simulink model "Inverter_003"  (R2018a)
settings: Solver=FixedStepDiscrete  StartTime=0.0  StopTime=inf  RelTol=1e-3  EnableMultiTasking=on
PreLoadFcn:
  | Sample_Time
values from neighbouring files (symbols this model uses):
  C_filt = 4.7e-6 /2  /2    (= 1.175e-06)    [Sample_Time.m]
  L_filt = 10e-3  /2  *2    (= 0.01)    [Sample_Time.m]
  Tcontrol = 5e-5    (= 5e-05)    [Sample_Time.m]
  Tmeasure = 5e-5     *2    (= 0.0001)    [Sample_Time.m]
  Tsample = 1e-6    (= 1e-06)    [Sample_Time.m]
  Tscope = Tcontrol*20    (= 0.001)    [Sample_Time.m]
  w = 2*pi*50    (= 314.159265359)    [Sample_Time.m]
undefined symbols (not defined in the file or in its folder): A, ADCIN0, ADCIN1, ADCINA0, ADCINB0, bit, C_filtEST, Compare, conversion, DCAEVT1, DCAEVT1FILT, Digital, Down, ended, Event, Filtered, GPTRIP1SEL, GPTRIP2SEL, input, Module, of, Single, start, Trip, TZ1, TZ2, Up, version, Zone
libraries: tiiqmathlib x32, simulink x16, c2802xlib x13, c2837xDlib x13, powerlib_meascontrol x4, etargetslib x4, c28xdmclib x1
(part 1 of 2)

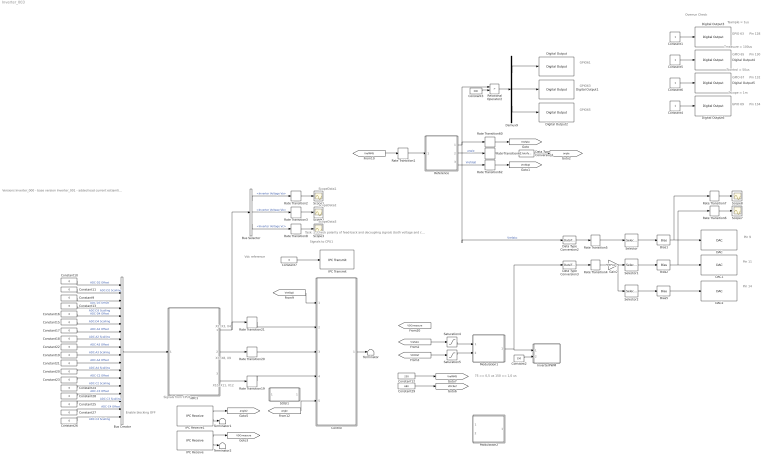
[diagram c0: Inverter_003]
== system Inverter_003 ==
  note: X2, X3, X4
  note: ScopeData3
  note: ScopeData2
  note: ScopeData1
  note: Vdc reference
  note: Enable blocking OFF
  note: Versions Inverter_000 - base version Inverter_001 - added load current estiamtion in control block Inverter_002 - PIR controller same as in PhD simulations Inverter_003 - Major changes to scaling and control blocks
  note: Task: 1. Check polarity of feed-back and decoupling signals (both voltage and current control)
  note: 75 == 0,5 us 150 == 1,0 us
  note: GPIO61
  note: GPIO63
  note: GPIO65
  note: Tcontrol = 50us
  note: GPIO 63
  note: Overrun Check
  note: Pin 128
  note: GPIO 69
  note: Pin 130
  note: Pin 134
  note: Pin 132
  note: GPIO 65
  note: Tsample = 1us
  note: Tmeasure = 100us
  note: Tscope = 1m
  note: GPIO 67
  note: Pin 14
  note: Pin 9
  note: Pin 11
  note: Signals from CPU1
  note: Signals to CPU1
  note: X7, X8, X9
  note: X10, X11, X12
  ADC1 : Subsystem
  Bias1 : Bias  Bias=400
  Bias2 : Bias  Bias=400
  Bias5 : Bias  Bias=400
  Bus Creator : BusCreator  Inputs=18
  Bus Selector : BusSelector  OutputSignals=Inverter Voltage Va,Inverter Voltage Vb,Inverter Voltage Vc
  Constant1 : Constant  Commented=on  SampleTime=Tsample
  Constant{9..11,13,15..28} (18 alike) : Constant  Value=0  OutDataTypeStr=single  SampleTime=0.1
  Constant12 : Constant  Value=230  OutDataTypeStr=single  SampleTime=0.1
  Constant2 : Constant  Value=150  OutDataTypeStr=single  SampleTime=0.1
  Constant29 : Constant  Value=680  OutDataTypeStr=fixdt(1,32,2^-10,0)  SampleTime=0.1
  Constant3 : Constant  Value=300  OutDataTypeStr=fixdt(1,32,2^-10,0)  SampleTime=0.1
  Constant4 : Constant  SampleTime=Tscope
  Constant5 : Constant  SampleTime=Tmeasure
  Constant6 : Constant  SampleTime=Tcontrol
  Constant7 : Constant  Value=0  OutDataTypeStr=single  SampleTime=Tcontrol
  Control : Subsystem  Commented=on
  DAC : c2837xDlib/DAC  channel=A  saturate=off
  DAC1 : c2837xDlib/DAC  channel=B  saturate=off
  DAC2 : c2837xDlib/DAC  channel=C  saturate=off
  Data Type Conversion1 : DataTypeConversion  OutDataTypeStr=single
  Data Type Conversion2 : DataTypeConversion  OutDataTypeStr=single
  Data Type Conversion3 : DataTypeConversion  OutDataTypeStr=single
  Demux9 : Demux  Outputs=3
  Digital Output : c2837xDlib/Digital Output  GPIO_Number=GPIO56~GPIO63  GPIO_Bit0=off  GPIO_BIT0_Toggle=off  GPIO_Bit1=off  GPIO_BIT1_Toggle=off  GPIO_Bit2=off  GPIO_BIT2_Toggle=off  GPIO_Bit3=off  GPIO_BIT3_Toggle=off  GPIO_Bit4=off  GPIO_BIT4_Toggle=off  GPIO_Bit5=on  GPIO_BIT5_Toggle=off  GPIO_Bit6=off  GPIO_BIT6_Toggle=off  GPIO_Bit7=off  GPIO_BIT7_Toggle=off
  Digital Output1 : c2837xDlib/Digital Output  GPIO_Number=GPIO56~GPIO63  GPIO_Bit0=off  GPIO_BIT0_Toggle=off  GPIO_Bit1=off  GPIO_BIT1_Toggle=off  GPIO_Bit2=off  GPIO_BIT2_Toggle=off  GPIO_Bit3=off  GPIO_BIT3_Toggle=off  GPIO_Bit4=off  GPIO_BIT4_Toggle=off  GPIO_Bit5=off  GPIO_BIT5_Toggle=off  GPIO_Bit6=off  GPIO_BIT6_Toggle=off  GPIO_Bit7=on  GPIO_BIT7_Toggle=off
  Digital Output2 : c2837xDlib/Digital Output  GPIO_Number=GPIO64~GPIO71  GPIO_Bit0=off  GPIO_BIT0_Toggle=off  GPIO_Bit1=off  GPIO_BIT1_Toggle=off  GPIO_Bit2=on  GPIO_BIT2_Toggle=off  GPIO_Bit3=off  GPIO_BIT3_Toggle=off  GPIO_Bit4=off  GPIO_BIT4_Toggle=off  GPIO_Bit5=off  GPIO_BIT5_Toggle=off  GPIO_Bit6=off  GPIO_BIT6_Toggle=off  GPIO_Bit7=off  GPIO_BIT7_Toggle=off
  Digital Output3 : c2837xDlib/Digital Output  Commented=on  GPIO_Number=GPIO56~GPIO63  GPIO_Bit0=off  GPIO_BIT0_Toggle=on  GPIO_Bit1=off  GPIO_BIT1_Toggle=off  GPIO_Bit2=off  GPIO_BIT2_Toggle=on  GPIO_Bit3=off  GPIO_BIT3_Toggle=off  GPIO_Bit4=off  GPIO_BIT4_Toggle=off  GPIO_Bit5=off  GPIO_BIT5_Toggle=off  GPIO_Bit6=off  GPIO_BIT6_Toggle=off  GPIO_Bit7=on  GPIO_BIT7_Toggle=on
  Digital Output4 : c2837xDlib/Digital Output  GPIO_Number=GPIO64~GPIO71  GPIO_Bit0=off  GPIO_BIT0_Toggle=on  GPIO_Bit1=on  GPIO_BIT1_Toggle=on  GPIO_Bit2=off  GPIO_BIT2_Toggle=on  GPIO_Bit3=off  GPIO_BIT3_Toggle=off  GPIO_Bit4=off  GPIO_BIT4_Toggle=off  GPIO_Bit5=off  GPIO_BIT5_Toggle=off  GPIO_Bit6=off  GPIO_BIT6_Toggle=off  GPIO_Bit7=off  GPIO_BIT7_Toggle=off
  Digital Output5 : c2837xDlib/Digital Output  GPIO_Number=GPIO64~GPIO71  GPIO_Bit0=off  GPIO_BIT0_Toggle=off  GPIO_Bit1=off  GPIO_BIT1_Toggle=off  GPIO_Bit2=off  GPIO_BIT2_Toggle=on  GPIO_Bit3=on  GPIO_BIT3_Toggle=on  GPIO_Bit4=off  GPIO_BIT4_Toggle=off  GPIO_Bit5=off  GPIO_BIT5_Toggle=off  GPIO_Bit6=off  GPIO_BIT6_Toggle=off  GPIO_Bit7=off  GPIO_BIT7_Toggle=off
  Digital Output6 : c2837xDlib/Digital Output  GPIO_Number=GPIO64~GPIO71  GPIO_Bit0=off  GPIO_BIT0_Toggle=on  GPIO_Bit1=off  GPIO_BIT1_Toggle=off  GPIO_Bit2=off  GPIO_BIT2_Toggle=on  GPIO_Bit3=off  GPIO_BIT3_Toggle=on  GPIO_Bit4=off  GPIO_BIT4_Toggle=off  GPIO_Bit5=on  GPIO_BIT5_Toggle=on  GPIO_Bit6=off  GPIO_BIT6_Toggle=off  GPIO_Bit7=off  GPIO_BIT7_Toggle=off
  Gain2 : Gain  Gain=230*sqrt(2)
  IPC Receive : c2837xDlib/IPC Receive  SelectChannel=0  DataType=single  DataLength=1  EnableBlocking=off  SampleTime=Tcontrol
  IPC Receive1 : c2837xDlib/IPC Receive  SelectChannel=2  DataType=single  DataLength=1  EnableBlocking=off  SampleTime=Tcontrol
  IPC Transmit : c2837xDlib/IPC Transmit  SelectChannel=1  EnableBlocking=off
  InverterPWM : Subsystem
  Modulation1 : Subsystem
  Modulation2 : Subsystem  Commented=on
  Rate Transition1 : RateTransition  OutPortSampleTime=10e-5
  Rate Transition{4..5,19..21,60..62} (8 alike) : RateTransition  OutPortSampleTime=Tcontrol
  Rate Transition2 : RateTransition  OutPortSampleTime=Tscope
  Rate Transition3 : RateTransition  OutPortSampleTime=Tscope
  Rate Transition6 : RateTransition  Commented=on  OutPortSampleTime=Tscope
  Rate Transition7 : RateTransition  Commented=on  OutPortSampleTime=Tscope
  Rate Transition8 : RateTransition  OutPortSampleTime=Tscope
  Reference : Subsystem  Commented=on
  Relational Operator2 : RelationalOperator  Operator=>  OutDataTypeStr=boolean
  SOGI1 : Subsystem  Commented=on  TreatAsAtomicUnit=on  mask{Freq=50, SampleTime=Tcontrol, UpperLimit=1000, LowerLimit=-1000}
      mask prompts: Freq "Frequency, Hz"; SampleTime "Sample Time, s"; UpperLimit "Upper Limit"; LowerLimit "Lower Limit"
  Saturation4 : Saturate  UpperLimit=400  LowerLimit=-400
  Saturation5 : Saturate  UpperLimit=720  LowerLimit=0
  Scope{1..3,7..8} (5 alike) : Scope
  Selector : Selector  InputPortWidth=3  IndexOptions=Index vector (dialog)  Indices=[2]  OutputSizes=1
  Selector1 : Selector  InputPortWidth=4  IndexOptions=Index vector (dialog)  Indices=[2]  OutputSizes=1
  Selector2 : Selector  InputPortWidth=4  IndexOptions=Index vector (dialog)  Indices=[4]  OutputSizes=1
  Terminator : Terminator
  Terminator1 : Terminator
  Terminator2 : Terminator
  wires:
  [Vrefabc] -> Saturation4/1
  [angle] -> Control/5(Angle)
  Constant2/1 -> InverterPWM/2(DeadBand)
  Saturation4/1 -> Modulation1/1(Vcontrol)
  Modulation1/1(VPWM) -> Data Type Conversion3/1, InverterPWM/1(PWM)
  Saturation5/1 -> Modulation1/2(VDC)
  Rate Transition21/1 -> Control/2(Vabc Phase)
  [Vrefdq0] -> Control/1(dq0Ref)
  [VDCRef] -> Saturation5/1
  Control/1(Vabc Control) -> Terminator/1
  Rate Transition20/1 -> Control/3(Iabc Inv)
  Rate Transition19/1 -> Control/4(Iabc Load)
  Demux9/2 -> Digital Output1/1
  Rate Transition1/1 -> Reference/1(Vac Ref)
  [VrefRMS] -> Rate Transition1/1
  Rate Transition61/1 -> Data Type Conversion1/1
  Reference/3(dq0) -> Rate Transition62/1  "Vrefdq0"
  Rate Transition62/1 -> [Vrefdq0]
  Reference/1(abc) -> Data Type Conversion2/1, Relational Operator2/1, Rate Transition60/1  "Vrefabc"
  Demux9/3 -> Digital Output2/1
  Reference/2(angle) -> Rate Transition61/1  "angle"
  Rate Transition60/1 -> [Vrefabc]
  Demux9/1 -> Digital Output/1
  Relational Operator2/1 -> Demux9/1
  Constant3/1 -> Relational Operator2/2
  Rate Transition4/1 -> Gain2/1
  Rate Transition5/1 -> Selector/1
  Data Type Conversion2/1 -> Rate Transition5/1
  Data Type Conversion3/1 -> Rate Transition4/1
  Gain2/1 -> Selector2/1, Selector1/1
  Selector/1 -> Bias1/1
  Selector1/1 -> Bias2/1
  Bias1/1 -> Rate Transition7/1, DAC/1
  Bias2/1 -> DAC1/1, Rate Transition6/1
  Rate Transition6/1 -> Scope7/1
  Rate Transition7/1 -> Scope8/1
  IPC Receive/1 -> [VDCmeasure]
  Selector2/1 -> Bias5/1
  Bias5/1 -> DAC2/1
  Constant7/1 -> IPC Transmit/1
  Constant6/1 -> Digital Output5/1
  Constant4/1 -> Digital Output6/1
  Constant5/1 -> Digital Output4/1
  Constant1/1 -> Digital Output3/1
  IPC Receive1/1 -> [angle2]
  Constant10/1 -> Bus Creator/1  "ADC-D2 Offset"
  Constant11/1 -> Bus Creator/2  "ADC-D2 Scalling"
  Constant13/1 -> Bus Creator/4  "ADC-D3 Scalling"
  Constant9/1 -> Bus Creator/3  "ADC-D3 Offset"
  Constant16/1 -> Bus Creator/5  "ADC-D4 Offset"
  Constant15/1 -> Bus Creator/6  "ADC-D4 Scalling"
  Constant20/1 -> Bus Creator/12  "ADC-A4 Scalling"
  Constant21/1 -> Bus Creator/11  "ADC-A4 Offset"
  Constant22/1 -> Bus Creator/9  "ADC-A3 Offset"
  Constant19/1 -> Bus Creator/10  "ADC-A3 Scalling"
  Constant18/1 -> Bus Creator/8  "ADC-A2 Scalling"
  Constant17/1 -> Bus Creator/7  "ADC-A2 Offset"
  Constant26/1 -> Bus Creator/18  "ADC-C4 Scalling"
  Constant27/1 -> Bus Creator/17  "ADC-C4 Offset"
  Constant28/1 -> Bus Creator/15  "ADC-C3 Offset"
  Constant25/1 -> Bus Creator/16  "ADC-C3 Scalling"
  Constant24/1 -> Bus Creator/14  "ADC-C2 Scalling"
  Constant23/1 -> Bus Creator/13  "ADC-C2 Offset"
  Bus Creator/1 -> ADC1/1(Scaling and Offset)
  ADC1/1(Inverter Voltage) -> Bus Selector/1, Rate Transition21/1
  ADC1/2(Inverter Current) -> Rate Transition20/1
  ADC1/3(Load Current) -> Rate Transition19/1
  Constant12/1 -> [VrefRMS]
  Constant29/1 -> [VDCRef]
  Rate Transition2/1 -> Scope1/1
  Bus Selector/1 -> Rate Transition2/1  "<Inverter Voltage Va>"
  Rate Transition3/1 -> Scope2/1
  Rate Transition8/1 -> Scope3/1
  Bus Selector/3 -> Rate Transition8/1  "<Inverter Voltage Vc>"
  Bus Selector/2 -> Rate Transition3/1  "<Inverter Voltage Vb>"
  IPC Receive1/2 -> Terminator1/1
  IPC Receive/2 -> Terminator2/1
  Data Type Conversion1/1 -> [angle]

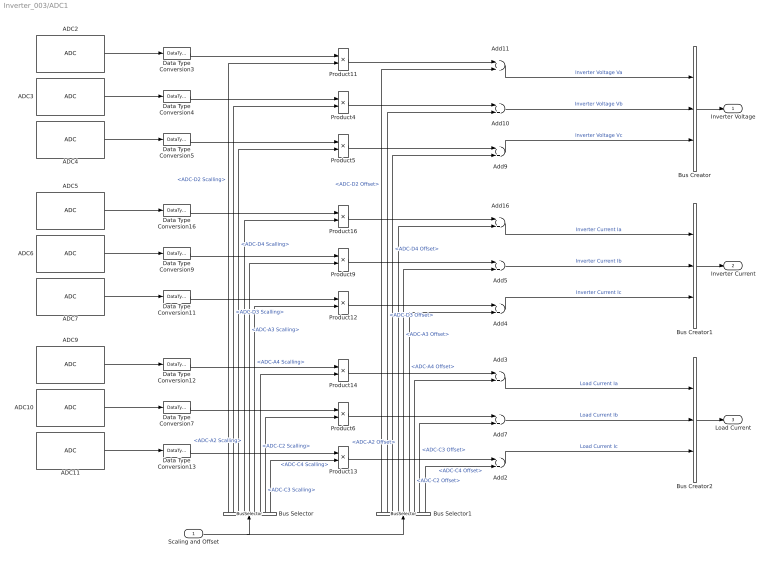
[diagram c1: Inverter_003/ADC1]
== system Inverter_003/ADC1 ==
  Scaling and Offset : Inport
  ADC10 : c2802xlib/ADC  blkParamProc=C2000_Type4  ADCModule=C  samplingMode=Single sample mode  ADCResolution=12-bit (Single-ended input)  useSOC1=SOC11  useSOC2=SOC0_SOC1  SOCAcquisitionWindow=15  SOCTriggerSource=Software  SOCInterruptTrigger=ADCINT1  Ts=Tmeasure  dType=uint16  postInterrupt=off  interruptSel=ADCINT1  ADCINTContinuous=on  endma=off  chdma=1  conv1=ADCINA0  conv2=ADCINA0 and ADCINB0  conv1_Type4=ADCIN3  conv2_Type4=ADCIN0 and ADCIN1
  ADC11 : c2802xlib/ADC  blkParamProc=C2000_Type4  ADCModule=C  samplingMode=Single sample mode  ADCResolution=12-bit (Single-ended input)  useSOC1=SOC12  useSOC2=SOC0_SOC1  SOCAcquisitionWindow=15  SOCTriggerSource=Software  SOCInterruptTrigger=ADCINT1  Ts=Tmeasure  dType=uint16  postInterrupt=off  interruptSel=ADCINT1  ADCINTContinuous=on  endma=off  chdma=1  conv1=ADCINA0  conv2=ADCINA0 and ADCINB0  conv1_Type4=ADCIN4  conv2_Type4=ADCIN0 and ADCIN1
  ADC2 : c2802xlib/ADC  blkParamProc=C2000_Type4  ADCModule=D  samplingMode=Single sample mode  ADCResolution=12-bit (Single-ended input)  useSOC1=SOC2  useSOC2=SOC0_SOC1  SOCAcquisitionWindow=15  SOCTriggerSource=Software  SOCInterruptTrigger=ADCINT1  Ts=Tmeasure  dType=uint16  postInterrupt=off  interruptSel=ADCINT1  ADCINTContinuous=on  endma=off  chdma=1  conv1=ADCINA0  conv2=ADCINA0 and ADCINB0  conv1_Type4=ADCIN2  conv2_Type4=ADCIN0 and ADCIN1
  ADC3 : c2802xlib/ADC  blkParamProc=C2000_Type4  ADCModule=D  samplingMode=Single sample mode  ADCResolution=12-bit (Single-ended input)  useSOC1=SOC5  useSOC2=SOC0_SOC1  SOCAcquisitionWindow=15  SOCTriggerSource=Software  SOCInterruptTrigger=ADCINT1  Ts=Tmeasure  dType=uint16  postInterrupt=off  interruptSel=ADCINT1  ADCINTContinuous=on  endma=off  chdma=1  conv1=ADCINA0  conv2=ADCINA0 and ADCINB0  conv1_Type4=ADCIN3  conv2_Type4=ADCIN0 and ADCIN1
  ADC4 : c2802xlib/ADC  blkParamProc=C2000_Type4  ADCModule=D  samplingMode=Single sample mode  ADCResolution=12-bit (Single-ended input)  useSOC1=SOC7  useSOC2=SOC0_SOC1  SOCAcquisitionWindow=15  SOCTriggerSource=Software  SOCInterruptTrigger=ADCINT1  Ts=Tmeasure  dType=uint16  postInterrupt=off  interruptSel=ADCINT1  ADCINTContinuous=on  endma=off  chdma=1  conv1=ADCINA0  conv2=ADCINA0 and ADCINB0  conv1_Type4=ADCIN4  conv2_Type4=ADCIN0 and ADCIN1
  ADC5 : c2802xlib/ADC  blkParamProc=C2000_Type4  ADCModule=A  samplingMode=Single sample mode  ADCResolution=12-bit (Single-ended input)  useSOC1=SOC4  useSOC2=SOC0_SOC1  SOCAcquisitionWindow=15  SOCTriggerSource=Software  SOCInterruptTrigger=ADCINT1  Ts=Tmeasure  dType=uint16  postInterrupt=off  interruptSel=ADCINT1  ADCINTContinuous=on  endma=off  chdma=1  conv1=ADCINA0  conv2=ADCINA0 and ADCINB0  conv1_Type4=ADCIN2  conv2_Type4=ADCIN0 and ADCIN1
  ADC6 : c2802xlib/ADC  blkParamProc=C2000_Type4  ADCModule=A  samplingMode=Single sample mode  ADCResolution=12-bit (Single-ended input)  useSOC1=SOC6  useSOC2=SOC0_SOC1  SOCAcquisitionWindow=15  SOCTriggerSource=Software  SOCInterruptTrigger=ADCINT1  Ts=Tmeasure  dType=uint16  postInterrupt=off  interruptSel=ADCINT1  ADCINTContinuous=on  endma=off  chdma=1  conv1=ADCINA0  conv2=ADCINA0 and ADCINB0  conv1_Type4=ADCIN3  conv2_Type4=ADCIN0 and ADCIN1
  ADC7 : c2802xlib/ADC  blkParamProc=C2000_Type4  ADCModule=A  samplingMode=Single sample mode  ADCResolution=12-bit (Single-ended input)  useSOC1=SOC8  useSOC2=SOC0_SOC1  SOCAcquisitionWindow=15  SOCTriggerSource=Software  SOCInterruptTrigger=ADCINT1  Ts=Tmeasure  dType=uint16  postInterrupt=off  interruptSel=ADCINT1  ADCINTContinuous=on  endma=off  chdma=1  conv1=ADCINA0  conv2=ADCINA0 and ADCINB0  conv1_Type4=ADCIN4  conv2_Type4=ADCIN0 and ADCIN1
  ADC9 : c2802xlib/ADC  blkParamProc=C2000_Type4  ADCModule=C  samplingMode=Single sample mode  ADCResolution=12-bit (Single-ended input)  useSOC1=SOC10  useSOC2=SOC0_SOC1  SOCAcquisitionWindow=15  SOCTriggerSource=Software  SOCInterruptTrigger=ADCINT1  Ts=Tmeasure  dType=uint16  postInterrupt=off  interruptSel=ADCINT1  ADCINTContinuous=on  endma=off  chdma=1  conv1=ADCINA0  conv2=ADCINA0 and ADCINB0  conv1_Type4=ADCIN2  conv2_Type4=ADCIN0 and ADCIN1
  Add{2..5,7,9..11,16} (9 alike) : Sum
  Bus Creator : BusCreator  Inputs=3
  Bus Creator1 : BusCreator  Inputs=3
  Bus Creator2 : BusCreator  Inputs=3
  Bus Selector : BusSelector  OutputSignals=ADC-D2 Scalling,ADC-D3 Scalling,ADC-D4 Scalling,ADC-A2 Scalling,ADC-A3 Scalling,ADC-A4 Scalling,ADC-C2 Scalling,ADC-C3 Scalling,ADC-C4 Scalling
  Bus Selector1 : BusSelector  OutputSignals=ADC-D2 Offset,ADC-D3 Offset,ADC-D4 Offset,ADC-A2 Offset,ADC-A3 Offset,ADC-A4 Offset,ADC-C2 Offset,ADC-C3 Offset,ADC-C4 Offset
  Data Type Conversion{3..5,7,9,11..13,16} (9 alike) : DataTypeConversion  OutDataTypeStr=single
  Product{4..6,9,11..14,16} (9 alike) : Product
  Inverter Voltage : Outport
  Inverter Current : Outport  Port=2
  Load Current : Outport  Port=3
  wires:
  ADC5/1 -> Data Type Conversion16/1
  ADC9/1 -> Data Type Conversion12/1
  ADC11/1 -> Data Type Conversion13/1
  ADC6/1 -> Data Type Conversion9/1
  ADC10/1 -> Data Type Conversion7/1
  ADC3/1 -> Data Type Conversion4/1
  ADC7/1 -> Data Type Conversion11/1
  ADC2/1 -> Data Type Conversion3/1
  ADC4/1 -> Data Type Conversion5/1
  Product11/1 -> Add11/1
  Data Type Conversion3/1 -> Product11/1
  Data Type Conversion4/1 -> Product4/1
  Data Type Conversion5/1 -> Product5/1
  Data Type Conversion16/1 -> Product16/1
  Data Type Conversion9/1 -> Product9/1
  Data Type Conversion11/1 -> Product12/1
  Data Type Conversion12/1 -> Product14/1
  Data Type Conversion7/1 -> Product6/1
  Data Type Conversion13/1 -> Product13/1
  Product13/1 -> Add2/1
  Product6/1 -> Add7/1
  Product14/1 -> Add3/1
  Product12/1 -> Add4/1
  Product9/1 -> Add5/1
  Product16/1 -> Add16/1
  Product5/1 -> Add9/1
  Product4/1 -> Add10/1
  Add11/1 -> Bus Creator/1  "Inverter Voltage Va"
  Add10/1 -> Bus Creator/2  "Inverter Voltage Vb"
  Add9/1 -> Bus Creator/3  "Inverter Voltage Vc"
  Add16/1 -> Bus Creator1/1  "Inverter Current Ia"
  Add5/1 -> Bus Creator1/2  "Inverter Current Ib"
  Add4/1 -> Bus Creator1/3  "Inverter Current Ic"
  Add3/1 -> Bus Creator2/1  "Load Current Ia"
  Add7/1 -> Bus Creator2/2  "Load Current Ib"
  Add2/1 -> Bus Creator2/3  "Load Current Ic"
  Scaling and Offset/1 -> Bus Selector/1, Bus Selector1/1
  Bus Selector/1 -> Product11/2  "<ADC-D2 Scalling>"
  Bus Selector/2 -> Product4/2  "<ADC-D3 Scalling>"
  Bus Selector/3 -> Product5/2  "<ADC-D4 Scalling>"
  Bus Selector/4 -> Product16/2  "<ADC-A2 Scalling>"
  Bus Selector/5 -> Product9/2  "<ADC-A3 Scalling>"
  Bus Selector/6 -> Product12/2  "<ADC-A4 Scalling>"
  Bus Selector/7 -> Product14/2  "<ADC-C2 Scalling>"
  Bus Selector/8 -> Product6/2  "<ADC-C3 Scalling>"
  Bus Selector/9 -> Product13/2  "<ADC-C4 Scalling>"
  Bus Selector1/9 -> Add2/2  "<ADC-C4 Offset>"
  Bus Selector1/8 -> Add7/2  "<ADC-C3 Offset>"
  Bus Selector1/6 -> Add4/2  "<ADC-A4 Offset>"
  Bus Selector1/7 -> Add3/2  "<ADC-C2 Offset>"
  Bus Selector1/5 -> Add5/2  "<ADC-A3 Offset>"
  Bus Selector1/4 -> Add16/2  "<ADC-A2 Offset>"
  Bus Selector1/3 -> Add9/2  "<ADC-D4 Offset>"
  Bus Selector1/2 -> Add10/2  "<ADC-D3 Offset>"
  Bus Selector1/1 -> Add11/2  "<ADC-D2 Offset>"
  Bus Creator/1 -> Inverter Voltage/1
  Bus Creator1/1 -> Inverter Current/1
  Bus Creator2/1 -> Load Current/1

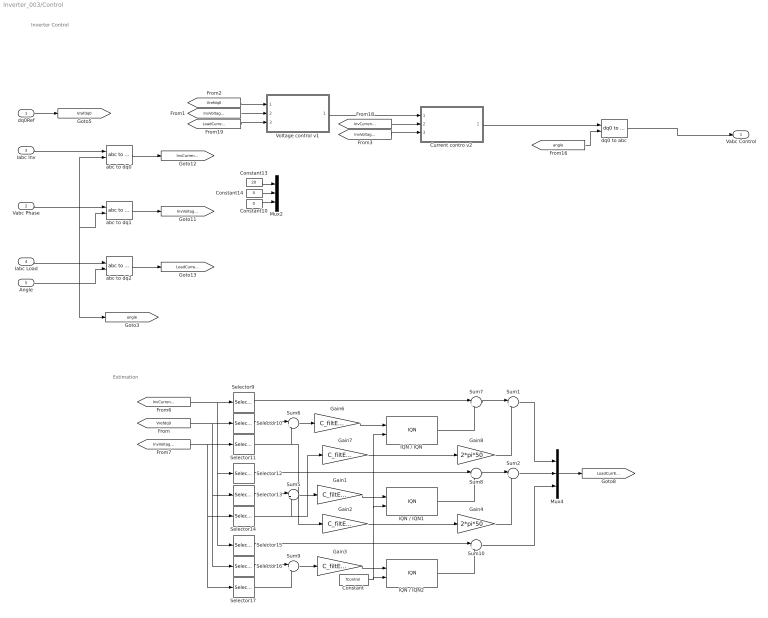
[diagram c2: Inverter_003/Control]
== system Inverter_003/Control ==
  note: Estimation
  note: Inverter Control
  dq0Ref : Inport
  Vabc Phase : Inport  Port=2
  Iabc Inv : Inport  Port=3
  Iabc Load : Inport  Port=4
  Angle : Inport  Port=5
  Constant : Constant  Commented=on  Value=Tcontrol
  Constant10 : Constant  Value=0  OutDataTypeStr=single  SampleTime=0.1
  Constant13 : Constant  Value=20  OutDataTypeStr=single  SampleTime=0.1
  Constant14 : Constant  Value=0  OutDataTypeStr=single  SampleTime=0.1
  Current contro v2 : Subsystem
  Gain{1..3,6..7} (5 alike) : Gain  Commented=on  Gain=C_filtEST
  Gain4 : Gain  Commented=on  Gain=2*pi*50
  Gain8 : Gain  Commented=on  Gain=2*pi*50
  IQN / IQN : tiiqmathlib/IQN // IQN  Commented=on
  IQN / IQN1 : tiiqmathlib/IQN // IQN  Commented=on
  IQN / IQN2 : tiiqmathlib/IQN // IQN  Commented=on
  Mux2 : Mux  Inputs=3
  Mux4 : Mux  Commented=on  Inputs=3
  Selector10 : Selector  Commented=on  InputPortWidth=3  IndexOptions=Index vector (dialog)  Indices=[1]  OutputSizes=1
  Selector11 : Selector  Commented=on  InputPortWidth=3  IndexOptions=Index vector (dialog)  Indices=[1]  OutputSizes=1
  Selector12 : Selector  Commented=on  InputPortWidth=3  IndexOptions=Index vector (dialog)  Indices=[2]  OutputSizes=1
  Selector13 : Selector  Commented=on  InputPortWidth=3  IndexOptions=Index vector (dialog)  Indices=[2]  OutputSizes=1
  Selector14 : Selector  Commented=on  InputPortWidth=3  IndexOptions=Index vector (dialog)  Indices=[2]  OutputSizes=1
  Selector15 : Selector  Commented=on  InputPortWidth=3  IndexOptions=Index vector (dialog)  Indices=[3]  OutputSizes=1
  Selector16 : Selector  Commented=on  InputPortWidth=3  IndexOptions=Index vector (dialog)  Indices=[3]  OutputSizes=1
  Selector17 : Selector  Commented=on  InputPortWidth=3  IndexOptions=Index vector (dialog)  Indices=[3]  OutputSizes=1
  Selector9 : Selector  Commented=on  InputPortWidth=3  IndexOptions=Index vector (dialog)  Indices=[1]  OutputSizes=1
  Sum1 : Sum  Commented=on  Inputs=|++
  Sum{2,5..10} (7 alike) : Sum  Commented=on  Inputs=|+-
  Voltage control v1 : Subsystem
  abc to dq0 : powerlib_meascontrol/Transformations/abc to dq0  Alignment=90 degrees behind phase A axis
  abc to dq1 : powerlib_meascontrol/Transformations/abc to dq0  Alignment=90 degrees behind phase A axis
  abc to dq2 : powerlib_meascontrol/Transformations/abc to dq0  Alignment=90 degrees behind phase A axis
  dq0 to abc : powerlib_meascontrol/Transformations/dq0 to abc  Alignment=90 degrees behind phase A axis
  Vabc Control : Outport
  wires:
  dq0 to abc/1 -> Vabc Control/1
  [LoadCurrentdq0] -> Voltage control v1/3(Id,q,0_load)
  [InvVoltagedq0] -> Current contro v2/3(Vd,q,0_load)
  Voltage control v1/1(Id,q,0_ref) -> Current contro v2/1(Id,q,0_ref)
  [angle] -> dq0 to abc/2
  Iabc Load/1 -> abc to dq2/1
  abc to dq2/1 -> [LoadCurrentdq0]
  abc to dq0/1 -> [InvCurrentdq0]
  abc to dq1/1 -> [InvVoltagedq0]
  Vabc Phase/1 -> abc to dq1/1
  Iabc Inv/1 -> abc to dq0/1
  [InvCurrentdq0] -> Current contro v2/2(Id,q,0)
  Angle/1 -> abc to dq2/2, abc to dq0/2, abc to dq1/2, [angle]
  dq0Ref/1 -> [Vrefdq0]
  Constant13/1 -> Mux2/1
  Constant14/1 -> Mux2/2
  Current contro v2/1(Vd,q,0_PWM) -> dq0 to abc/1
  [Vrefdq0] -> Voltage control v1/1(Vd,q,0_ref)
  Constant10/1 -> Mux2/3
  Mux4/1 -> [LoadCurrEstdq0]
  Sum8/1 -> Sum2/1
  Gain8/1 -> Sum1/2
  Gain7/1 -> Gain8/1
  Gain2/1 -> Gain4/1
  Gain4/1 -> Sum2/2
  Sum7/1 -> Sum1/1
  Sum10/1 -> Mux4/3
  Sum2/1 -> Mux4/2
  Sum1/1 -> Mux4/1
  Selector17/1 -> Sum9/2
  Sum9/1 -> Gain3/1
  IQN / IQN2/1 -> Sum10/2
  Gain3/1 -> IQN / IQN2/1
  Selector15/1 -> Sum10/1
  Selector16/1 -> Sum9/1
  Selector14/1 -> Sum5/2, Gain7/1
  Sum5/1 -> Gain1/1
  IQN / IQN1/1 -> Sum8/2
  Gain1/1 -> IQN / IQN1/1
  Selector12/1 -> Sum8/1
  Selector13/1 -> Sum5/1
  [InvVoltagedq0] -> Selector14/1, Selector17/1, Selector11/1
  [Vrefdq0] -> Selector16/1, Selector13/1, Selector10/1
  [InvCurrentdq0] -> Selector12/1, Selector15/1, Selector9/1
  Selector11/1 -> Sum6/2, Gain2/1
  Sum6/1 -> Gain6/1
  IQN / IQN/1 -> Sum7/2
  Gain6/1 -> IQN / IQN/1
  Selector9/1 -> Sum7/1
  Selector10/1 -> Sum6/1
  Constant/1 -> IQN / IQN1/2, IQN / IQN/2, IQN / IQN2/2
  [InvVoltagedq0] -> Voltage control v1/2(Vd,q,0_load)

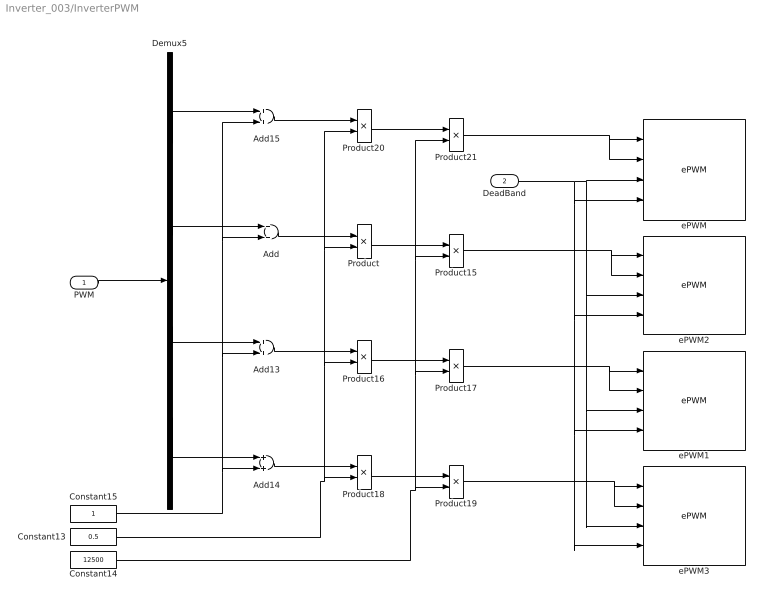
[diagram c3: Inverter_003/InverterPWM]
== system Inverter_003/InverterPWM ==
  PWM : Inport
  DeadBand : Inport  Port=2
  Add{,13..15} (4 alike) : Sum
  Constant13 : Constant  Value=0.5  OutDataTypeStr=single  SampleTime=0.1
  Constant14 : Constant  Value=12500  OutDataTypeStr=single  SampleTime=0.1
  Constant15 : Constant  OutDataTypeStr=single  SampleTime=0.1
  Demux5 : Demux
  Product{,15..21} (8 alike) : Product
  ePWM : c2802xlib/ePWM  useModule=ePWM5  ePWMxLINKTBPRD=Not Linked  periodUnits=Clock cycles  timerSource=Specify via dialog  timerPeriod_clk=12500  timerPeriod_sec=0.0001  tbshadow=Counter equals to zero  countingMode=Up-Down  phaseActiveEnable=Disable  phaseDirection=Count down after sync  phaseActive=0  synchronizationEnable=off  dcaevt1Sync=off  dcbevt1Sync=off  synchronizationOption=Disable  clockPrescale=1  HSclockPrescale=1  enswap=off  ePWMxAStatus=on  ePWMxAactionLogic1=Set  ePWMxAactionLogic2=Clear  ePWMxAactionLogic3=Clear  ePWMxAactionLogic4=Set  ePWMxAactionLogic5=Do nothing  ePWMxAactionLogic6=Do nothing  ePWMxALoadMode=Load on counter equals to zero (CTR=Zero)  ePWMxACSFenable=off  ePWMxACSFvalue=Forcing disable  ePWMxASFreload=Zero  ePWMxBStatus=on  ePWMxBactionLogic1=Clear  ePWMxBactionLogic2=Set  ePWMxBactionLogic3=Do nothing  ePWMxBactionLogic4=Do nothing  ePWMxBactionLogic5=Set  ePWMxBactionLogic6=Clear  ePWMxBLoadMode=Load on counter equals to zero (CTR=Zero)  ePWMxBCSFenable=off  ePWMxBCSFvalue=Forcing disable  ePWMxBSFreload=Zero  ePWNxBOutWay=off  ePWMxLINKCMPA=Not Linked  CMPAUnits=Clock cycles  CMPASource=Input port  CMPAValue_per=50  CMPAValue_clk=3750  enCMPAshadow=Counter equals to zero  ePWMxLINKCMPB=Not Linked  CMPBUnits=Clock cycles  CMPBSource=Input port  CMPBValue_per=50  CMPBValue_clk=3750  enCMPBshadow=Counter equals to zero  ePWMxLINKCMPC=Not Linked  CMPCUnits=Clock cycles  CMPCSource=Specify via dialog  CMPCValue_per=50  CMPCValue_clk=32000  enCMPCshadow=Counter equals to zero  ePWMxLINKCMPD=Not Linked  CMPDUnits=Clock cycles  CMPDSource=Specify via dialog  CMPDValue_per=50  CMPDValue_clk=32000  enCMPDshadow=Counter equals to zero  enableDBePWMxA=on  enableDBePWMxB=on  enhalfcycle=off  DBpolarity=Active high complementary (AHC)  DBedgeDelay=Positive  DBSource_ePWMxA=ePWMxA  DBSource_ePWMxB=ePWMxA  DBperiodSource=Input port  REDperiod=0  FEDperiod=0  adcstartModuleA=off  adcrequestEventA=First event  adcstartEventA=Digital Compare Module A Event 1 start of conversion (DCAEVT1.soc)  adcstartEventA_type2=Digital Compare Module A Event 1 start of conversion (DCAEVT1.soc)  adcstartModuleB=off  adcrequestEventB=First event  adcstartEventB=Counter equals to zero (CTR=Zero)  adcstartEventB_type2=Counter equals to zero (CTR=Zero)  intEn=off  intPrd=First event  intSel=Counter equals to zero (CTR=Zero)  intSel_type2=Counter equals to zero (CTR=Zero)  hrpe=off  enHRPWM=off  HRPWM_LoadMode=Counter equals to period (CTR=PRD)  HRPWM_CTLMode=Duty or Period control mode  HRPWM_EDGMode=Both edge  hrpeb=off  enHRPWMB=off  HRPWM_LoadModeB=Counter equals to zero (CTR=ZERO)  HRPWM_CTLModeB=Duty or Period control mode  HRPWM_EDGModeB=Both edge  enSFO=on  enautoconv=on  chopperEnable=off  chopperFrequency=1  chopperFirstwidth=1  chopperDuty=12.5%  tripZonesource=Specify via dialog  tzselOSHT1=off  tzselOSHT2=off  tzselOSHT3=off  tzselOSHDCAEV1=off  tzselOSHDCBEV1=off  tzselCBC1=off  tzselCBC2=off  tzselCBC3=off  tzselCBCDCAEV2=off  tzselCBCDCBEV2=off  tzselOSHT4=off  tzselOSHT5=off  tzselOSHT6=off  tzselCBC4=off  tzselCBC5=off  tzselCBC6=off  enTzOstIntr=off  enTzCbcIntr=off  enTzDCAEVT1Intr=off  enTzDCAEVT2Intr=off  enTzDCBEVT1Intr=off  enTzDCBEVT2Intr=off  ePWMxAforced=No action  ePWMxBforced=No action  DCAEVT1forced=No action  DCBEVT1forced=No action  DCAEVT2forced=No action  DCBEVT2forced=No action  dcah=Trip Zone 1 input (TZ1)  dcal=Trip Zone 2 input (TZ2)  dcbh=Trip Zone 1 input (TZ1)  dcbl=Trip Zone 2 input (TZ2)  dcah_type2=GPTRIP1SEL/(TZ1)  dcal_type2=GPTRIP2SEL/(TZ2)  dcbh_type2=GPTRIP1SEL/(TZ1)  dcbl_type2=GPTRIP2SEL/(TZ2)  gendcaevt1=Event disabled  gendcaevt2=Event disabled  gendcbevt1=Event disabled  gendcbevt2=Event disabled  dcaevt1src=DCAEVT1 with sync  dcaevt2src=DCAEVT2 with sync  dcbevt1src=DCBEVT1 with sync  dcbevt2src=DCBEVT2 with sync  pulsesel=Counter equals to zero (CTR=Zero)  blankinv=off  blankoffset=0  blankwidth=0  evsrcsel=Filtered version of DCAEVT1 (DCAEVT1FILT)  encape=off  PwmType=C2000_Type4
  ePWM1 : c2802xlib/ePWM  useModule=ePWM3  ePWMxLINKTBPRD=Not Linked  periodUnits=Clock cycles  timerSource=Specify via dialog  timerPeriod_clk=12500  timerPeriod_sec=0.0001  tbshadow=Counter equals to zero  countingMode=Up-Down  phaseActiveEnable=Disable  phaseDirection=Count down after sync  phaseActive=0  synchronizationEnable=off  dcaevt1Sync=off  dcbevt1Sync=off  synchronizationOption=Disable  clockPrescale=1  HSclockPrescale=1  enswap=off  ePWMxAStatus=on  ePWMxAactionLogic1=Set  ePWMxAactionLogic2=Clear  ePWMxAactionLogic3=Clear  ePWMxAactionLogic4=Set  ePWMxAactionLogic5=Do nothing  ePWMxAactionLogic6=Do nothing  ePWMxALoadMode=Load on counter equals to zero (CTR=Zero)  ePWMxACSFenable=off  ePWMxACSFvalue=Forcing disable  ePWMxASFreload=Zero  ePWMxBStatus=on  ePWMxBactionLogic1=Clear  ePWMxBactionLogic2=Set  ePWMxBactionLogic3=Do nothing  ePWMxBactionLogic4=Do nothing  ePWMxBactionLogic5=Set  ePWMxBactionLogic6=Clear  ePWMxBLoadMode=Load on counter equals to zero (CTR=Zero)  ePWMxBCSFenable=off  ePWMxBCSFvalue=Forcing disable  ePWMxBSFreload=Zero  ePWNxBOutWay=off  ePWMxLINKCMPA=Not Linked  CMPAUnits=Clock cycles  CMPASource=Input port  CMPAValue_per=50  CMPAValue_clk=3750  enCMPAshadow=Counter equals to zero  ePWMxLINKCMPB=Not Linked  CMPBUnits=Clock cycles  CMPBSource=Input port  CMPBValue_per=50  CMPBValue_clk=3750  enCMPBshadow=Counter equals to zero  ePWMxLINKCMPC=Not Linked  CMPCUnits=Clock cycles  CMPCSource=Specify via dialog  CMPCValue_per=50  CMPCValue_clk=32000  enCMPCshadow=Counter equals to zero  ePWMxLINKCMPD=Not Linked  CMPDUnits=Clock cycles  CMPDSource=Specify via dialog  CMPDValue_per=50  CMPDValue_clk=32000  enCMPDshadow=Counter equals to zero  enableDBePWMxA=on  enableDBePWMxB=on  enhalfcycle=off  DBpolarity=Active high complementary (AHC)  DBedgeDelay=Positive  DBSource_ePWMxA=ePWMxA  DBSource_ePWMxB=ePWMxA  DBperiodSource=Input port  REDperiod=0  FEDperiod=0  adcstartModuleA=off  adcrequestEventA=First event  adcstartEventA=Digital Compare Module A Event 1 start of conversion (DCAEVT1.soc)  adcstartEventA_type2=Digital Compare Module A Event 1 start of conversion (DCAEVT1.soc)  adcstartModuleB=off  adcrequestEventB=First event  adcstartEventB=Counter equals to zero (CTR=Zero)  adcstartEventB_type2=Counter equals to zero (CTR=Zero)  intEn=off  intPrd=First event  intSel=Counter equals to zero (CTR=Zero)  intSel_type2=Counter equals to zero (CTR=Zero)  hrpe=off  enHRPWM=off  HRPWM_LoadMode=Counter equals to period (CTR=PRD)  HRPWM_CTLMode=Duty or Period control mode  HRPWM_EDGMode=Both edge  hrpeb=off  enHRPWMB=off  HRPWM_LoadModeB=Counter equals to zero (CTR=ZERO)  HRPWM_CTLModeB=Duty or Period control mode  HRPWM_EDGModeB=Both edge  enSFO=on  enautoconv=on  chopperEnable=off  chopperFrequency=1  chopperFirstwidth=1  chopperDuty=12.5%  tripZonesource=Specify via dialog  tzselOSHT1=off  tzselOSHT2=off  tzselOSHT3=off  tzselOSHDCAEV1=off  tzselOSHDCBEV1=off  tzselCBC1=off  tzselCBC2=off  tzselCBC3=off  tzselCBCDCAEV2=off  tzselCBCDCBEV2=off  tzselOSHT4=off  tzselOSHT5=off  tzselOSHT6=off  tzselCBC4=off  tzselCBC5=off  tzselCBC6=off  enTzOstIntr=off  enTzCbcIntr=off  enTzDCAEVT1Intr=off  enTzDCAEVT2Intr=off  enTzDCBEVT1Intr=off  enTzDCBEVT2Intr=off  ePWMxAforced=No action  ePWMxBforced=No action  DCAEVT1forced=No action  DCBEVT1forced=No action  DCAEVT2forced=No action  DCBEVT2forced=No action  dcah=Trip Zone 1 input (TZ1)  dcal=Trip Zone 2 input (TZ2)  dcbh=Trip Zone 1 input (TZ1)  dcbl=Trip Zone 2 input (TZ2)  dcah_type2=GPTRIP1SEL/(TZ1)  dcal_type2=GPTRIP2SEL/(TZ2)  dcbh_type2=GPTRIP1SEL/(TZ1)  dcbl_type2=GPTRIP2SEL/(TZ2)  gendcaevt1=Event disabled  gendcaevt2=Event disabled  gendcbevt1=Event disabled  gendcbevt2=Event disabled  dcaevt1src=DCAEVT1 with sync  dcaevt2src=DCAEVT2 with sync  dcbevt1src=DCBEVT1 with sync  dcbevt2src=DCBEVT2 with sync  pulsesel=Counter equals to zero (CTR=Zero)  blankinv=off  blankoffset=0  blankwidth=0  evsrcsel=Filtered version of DCAEVT1 (DCAEVT1FILT)  encape=off  PwmType=C2000_Type4
  ePWM2 : c2802xlib/ePWM  useModule=ePWM6  ePWMxLINKTBPRD=Not Linked  periodUnits=Clock cycles  timerSource=Specify via dialog  timerPeriod_clk=12500  timerPeriod_sec=0.0001  tbshadow=Counter equals to zero  countingMode=Up-Down  phaseActiveEnable=Disable  phaseDirection=Count down after sync  phaseActive=0  synchronizationEnable=off  dcaevt1Sync=off  dcbevt1Sync=off  synchronizationOption=Disable  clockPrescale=1  HSclockPrescale=1  enswap=off  ePWMxAStatus=on  ePWMxAactionLogic1=Set  ePWMxAactionLogic2=Clear  ePWMxAactionLogic3=Clear  ePWMxAactionLogic4=Set  ePWMxAactionLogic5=Do nothing  ePWMxAactionLogic6=Do nothing  ePWMxALoadMode=Load on counter equals to zero (CTR=Zero)  ePWMxACSFenable=off  ePWMxACSFvalue=Forcing disable  ePWMxASFreload=Zero  ePWMxBStatus=on  ePWMxBactionLogic1=Clear  ePWMxBactionLogic2=Set  ePWMxBactionLogic3=Do nothing  ePWMxBactionLogic4=Do nothing  ePWMxBactionLogic5=Set  ePWMxBactionLogic6=Clear  ePWMxBLoadMode=Load on counter equals to zero (CTR=Zero)  ePWMxBCSFenable=off  ePWMxBCSFvalue=Forcing disable  ePWMxBSFreload=Zero  ePWNxBOutWay=off  ePWMxLINKCMPA=Not Linked  CMPAUnits=Clock cycles  CMPASource=Input port  CMPAValue_per=50  CMPAValue_clk=3750  enCMPAshadow=Counter equals to zero  ePWMxLINKCMPB=Not Linked  CMPBUnits=Clock cycles  CMPBSource=Input port  CMPBValue_per=50  CMPBValue_clk=3750  enCMPBshadow=Counter equals to zero  ePWMxLINKCMPC=Not Linked  CMPCUnits=Clock cycles  CMPCSource=Specify via dialog  CMPCValue_per=50  CMPCValue_clk=32000  enCMPCshadow=Counter equals to zero  ePWMxLINKCMPD=Not Linked  CMPDUnits=Clock cycles  CMPDSource=Specify via dialog  CMPDValue_per=50  CMPDValue_clk=32000  enCMPDshadow=Counter equals to zero  enableDBePWMxA=on  enableDBePWMxB=on  enhalfcycle=off  DBpolarity=Active high complementary (AHC)  DBedgeDelay=Positive  DBSource_ePWMxA=ePWMxA  DBSource_ePWMxB=ePWMxA  DBperiodSource=Input port  REDperiod=0  FEDperiod=0  adcstartModuleA=off  adcrequestEventA=First event  adcstartEventA=Digital Compare Module A Event 1 start of conversion (DCAEVT1.soc)  adcstartEventA_type2=Digital Compare Module A Event 1 start of conversion (DCAEVT1.soc)  adcstartModuleB=off  adcrequestEventB=First event  adcstartEventB=Counter equals to zero (CTR=Zero)  adcstartEventB_type2=Counter equals to zero (CTR=Zero)  intEn=off  intPrd=First event  intSel=Counter equals to zero (CTR=Zero)  intSel_type2=Counter equals to zero (CTR=Zero)  hrpe=off  enHRPWM=off  HRPWM_LoadMode=Counter equals to period (CTR=PRD)  HRPWM_CTLMode=Duty or Period control mode  HRPWM_EDGMode=Both edge  hrpeb=off  enHRPWMB=off  HRPWM_LoadModeB=Counter equals to zero (CTR=ZERO)  HRPWM_CTLModeB=Duty or Period control mode  HRPWM_EDGModeB=Both edge  enSFO=on  enautoconv=on  chopperEnable=off  chopperFrequency=1  chopperFirstwidth=1  chopperDuty=12.5%  tripZonesource=Specify via dialog  tzselOSHT1=off  tzselOSHT2=off  tzselOSHT3=off  tzselOSHDCAEV1=off  tzselOSHDCBEV1=off  tzselCBC1=off  tzselCBC2=off  tzselCBC3=off  tzselCBCDCAEV2=off  tzselCBCDCBEV2=off  tzselOSHT4=off  tzselOSHT5=off  tzselOSHT6=off  tzselCBC4=off  tzselCBC5=off  tzselCBC6=off  enTzOstIntr=off  enTzCbcIntr=off  enTzDCAEVT1Intr=off  enTzDCAEVT2Intr=off  enTzDCBEVT1Intr=off  enTzDCBEVT2Intr=off  ePWMxAforced=No action  ePWMxBforced=No action  DCAEVT1forced=No action  DCBEVT1forced=No action  DCAEVT2forced=No action  DCBEVT2forced=No action  dcah=Trip Zone 1 input (TZ1)  dcal=Trip Zone 2 input (TZ2)  dcbh=Trip Zone 1 input (TZ1)  dcbl=Trip Zone 2 input (TZ2)  dcah_type2=GPTRIP1SEL/(TZ1)  dcal_type2=GPTRIP2SEL/(TZ2)  dcbh_type2=GPTRIP1SEL/(TZ1)  dcbl_type2=GPTRIP2SEL/(TZ2)  gendcaevt1=Event disabled  gendcaevt2=Event disabled  gendcbevt1=Event disabled  gendcbevt2=Event disabled  dcaevt1src=DCAEVT1 with sync  dcaevt2src=DCAEVT2 with sync  dcbevt1src=DCBEVT1 with sync  dcbevt2src=DCBEVT2 with sync  pulsesel=Counter equals to zero (CTR=Zero)  blankinv=off  blankoffset=0  blankwidth=0  evsrcsel=Filtered version of DCAEVT1 (DCAEVT1FILT)  encape=off  PwmType=C2000_Type4
  ePWM3 : c2802xlib/ePWM  useModule=ePWM4  ePWMxLINKTBPRD=Not Linked  periodUnits=Clock cycles  timerSource=Specify via dialog  timerPeriod_clk=12500  timerPeriod_sec=0.0001  tbshadow=Counter equals to zero  countingMode=Up-Down  phaseActiveEnable=Disable  phaseDirection=Count down after sync  phaseActive=0  synchronizationEnable=off  dcaevt1Sync=off  dcbevt1Sync=off  synchronizationOption=Disable  clockPrescale=1  HSclockPrescale=1  enswap=off  ePWMxAStatus=on  ePWMxAactionLogic1=Set  ePWMxAactionLogic2=Clear  ePWMxAactionLogic3=Clear  ePWMxAactionLogic4=Set  ePWMxAactionLogic5=Do nothing  ePWMxAactionLogic6=Do nothing  ePWMxALoadMode=Load on counter equals to zero (CTR=Zero)  ePWMxACSFenable=off  ePWMxACSFvalue=Forcing disable  ePWMxASFreload=Zero  ePWMxBStatus=on  ePWMxBactionLogic1=Clear  ePWMxBactionLogic2=Set  ePWMxBactionLogic3=Do nothing  ePWMxBactionLogic4=Do nothing  ePWMxBactionLogic5=Set  ePWMxBactionLogic6=Clear  ePWMxBLoadMode=Load on counter equals to zero (CTR=Zero)  ePWMxBCSFenable=off  ePWMxBCSFvalue=Forcing disable  ePWMxBSFreload=Zero  ePWNxBOutWay=off  ePWMxLINKCMPA=Not Linked  CMPAUnits=Clock cycles  CMPASource=Input port  CMPAValue_per=50  CMPAValue_clk=3750  enCMPAshadow=Counter equals to zero  ePWMxLINKCMPB=Not Linked  CMPBUnits=Clock cycles  CMPBSource=Input port  CMPBValue_per=50  CMPBValue_clk=3750  enCMPBshadow=Counter equals to zero  ePWMxLINKCMPC=Not Linked  CMPCUnits=Clock cycles  CMPCSource=Specify via dialog  CMPCValue_per=50  CMPCValue_clk=32000  enCMPCshadow=Counter equals to zero  ePWMxLINKCMPD=Not Linked  CMPDUnits=Clock cycles  CMPDSource=Specify via dialog  CMPDValue_per=50  CMPDValue_clk=32000  enCMPDshadow=Counter equals to zero  enableDBePWMxA=on  enableDBePWMxB=on  enhalfcycle=off  DBpolarity=Active high complementary (AHC)  DBedgeDelay=Positive  DBSource_ePWMxA=ePWMxA  DBSource_ePWMxB=ePWMxA  DBperiodSource=Input port  REDperiod=0  FEDperiod=0  adcstartModuleA=off  adcrequestEventA=First event  adcstartEventA=Digital Compare Module A Event 1 start of conversion (DCAEVT1.soc)  adcstartEventA_type2=Digital Compare Module A Event 1 start of conversion (DCAEVT1.soc)  adcstartModuleB=off  adcrequestEventB=First event  adcstartEventB=Counter equals to zero (CTR=Zero)  adcstartEventB_type2=Counter equals to zero (CTR=Zero)  intEn=off  intPrd=First event  intSel=Counter equals to zero (CTR=Zero)  intSel_type2=Counter equals to zero (CTR=Zero)  hrpe=off  enHRPWM=off  HRPWM_LoadMode=Counter equals to period (CTR=PRD)  HRPWM_CTLMode=Duty or Period control mode  HRPWM_EDGMode=Both edge  hrpeb=off  enHRPWMB=off  HRPWM_LoadModeB=Counter equals to zero (CTR=ZERO)  HRPWM_CTLModeB=Duty or Period control mode  HRPWM_EDGModeB=Both edge  enSFO=on  enautoconv=on  chopperEnable=off  chopperFrequency=1  chopperFirstwidth=1  chopperDuty=12.5%  tripZonesource=Specify via dialog  tzselOSHT1=off  tzselOSHT2=off  tzselOSHT3=off  tzselOSHDCAEV1=off  tzselOSHDCBEV1=off  tzselCBC1=off  tzselCBC2=off  tzselCBC3=off  tzselCBCDCAEV2=off  tzselCBCDCBEV2=off  tzselOSHT4=off  tzselOSHT5=off  tzselOSHT6=off  tzselCBC4=off  tzselCBC5=off  tzselCBC6=off  enTzOstIntr=off  enTzCbcIntr=off  enTzDCAEVT1Intr=off  enTzDCAEVT2Intr=off  enTzDCBEVT1Intr=off  enTzDCBEVT2Intr=off  ePWMxAforced=No action  ePWMxBforced=No action  DCAEVT1forced=No action  DCBEVT1forced=No action  DCAEVT2forced=No action  DCBEVT2forced=No action  dcah=Trip Zone 1 input (TZ1)  dcal=Trip Zone 2 input (TZ2)  dcbh=Trip Zone 1 input (TZ1)  dcbl=Trip Zone 2 input (TZ2)  dcah_type2=GPTRIP1SEL/(TZ1)  dcal_type2=GPTRIP2SEL/(TZ2)  dcbh_type2=GPTRIP1SEL/(TZ1)  dcbl_type2=GPTRIP2SEL/(TZ2)  gendcaevt1=Event disabled  gendcaevt2=Event disabled  gendcbevt1=Event disabled  gendcbevt2=Event disabled  dcaevt1src=DCAEVT1 with sync  dcaevt2src=DCAEVT2 with sync  dcbevt1src=DCBEVT1 with sync  dcbevt2src=DCBEVT2 with sync  pulsesel=Counter equals to zero (CTR=Zero)  blankinv=off  blankoffset=0  blankwidth=0  evsrcsel=Filtered version of DCAEVT1 (DCAEVT1FILT)  encape=off  PwmType=C2000_Type4
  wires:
  PWM/1 -> Demux5/1
  Product/1 -> Product15/1
  Add/1 -> Product/1
  Add14/1 -> Product18/1
  Add13/1 -> Product16/1
  Product18/1 -> Product19/1
  Product16/1 -> Product17/1
  Constant15/1 -> Add15/2, Add/2, Add13/2, Add14/2
  Product20/1 -> Product21/1
  Add15/1 -> Product20/1
  Constant14/1 -> Product17/2, Product21/2, Product15/2, Product19/2
  Constant13/1 -> Product18/2, Product16/2, Product20/2, Product/2
  Demux5/1 -> Add15/1
  Demux5/2 -> Add/1
  Demux5/3 -> Add13/1
  Demux5/4 -> Add14/1
  Product19/1 -> ePWM3/1, ePWM3/2
  Product15/1 -> ePWM2/1, ePWM2/2
  Product17/1 -> ePWM1/1, ePWM1/2
  Product21/1 -> ePWM/1, ePWM/2
  DeadBand/1 -> ePWM/4, ePWM2/4, ePWM3/4, ePWM1/4, ePWM/3, ePWM2/3, ePWM3/3, ePWM1/3

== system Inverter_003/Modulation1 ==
  Vcontrol : Inport
  VDC : Inport  Port=2
  Constant : Constant  Value=0.0  OutDataTypeStr=fixdt(1,32,2^-10,0)
  Float to IQN2 : tiiqmathlib/Float to IQN  Q_value=10
  Gain1 : Gain  Gain=0.5  OutDataTypeStr=single
  IQN / IQN : tiiqmathlib/IQN // IQN
  Mux : Mux  Inputs=2
  PPPWM_offset : Subsystem  TreatAsAtomicUnit=on  mask(PPPWM3){}
      mask help: PPPWM3 Input: 1 - size 4, reference phase waveforms [1-3] and DC bus voltage [4] Output: 1 - size 4, modulation waveforms for three-phase two-level four-leg inverter (a,b,c,n) Source: S.J. Chee, S. Ko, H.S. Kim and S.K. Sul, "Common-Mode Voltage Reduction of Three-Level Four-Leg PWM Converter", IEEE Transactions on Industry Applications, vol. 51, no. 5, Sept.-Oct. 2015, pp. 4006-4016
  Subsystem : Subsystem  TreatAsAtomicUnit=on
  VPWM : Outport
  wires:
  Vcontrol/1 -> Subsystem/1(Vref), Mux/1
  Mux/1 -> PPPWM_offset/1(In [4])
  Constant/1 -> PPPWM_offset/2(Offset)
  IQN / IQN/1 -> VPWM/1
  Float to IQN2/1 -> IQN / IQN/2
  Gain1/1 -> Float to IQN2/1
  VDC/1 -> Mux/2, Gain1/1
  Subsystem/1(Out[4]) -> IQN / IQN/1

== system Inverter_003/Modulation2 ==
  Vcontrol : Inport
  VDC : Inport  Port=2
  Add16 : Sum
  Add17 : Sum
  Add18 : Sum
  Carrier1 : Subsystem
  Demux4 : Demux  Outputs=3
  Float to IQN1 : tiiqmathlib/Float to IQN  Q_value=10
  Gain : Gain  Gain=0.5  OutDataTypeStr=single
  IQN / IQN : tiiqmathlib/IQN // IQN
  IQN / IQN1 : tiiqmathlib/IQN // IQN
  IQN / IQN2 : tiiqmathlib/IQN // IQN
  Mux6 : Mux
  Mux7 : Mux  Inputs=3
  VPWM : Outport
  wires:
  IQN / IQN/1 -> Add16/1, Mux7/1
  Float to IQN1/1 -> IQN / IQN2/2, IQN / IQN/2, IQN / IQN1/2
  Vcontrol/1 -> Demux4/1
  Gain/1 -> Float to IQN1/1
  IQN / IQN2/1 -> Add18/1, Mux7/3
  Add18/1 -> Mux6/3  "PhaseC"
  VDC/1 -> Gain/1
  Demux4/3 -> IQN / IQN2/1
  Mux6/1 -> VPWM/1
  Demux4/1 -> IQN / IQN/1
  IQN / IQN1/1 -> Add17/1, Mux7/2
  Mux7/1 -> Carrier1/1(In1)
  Add16/1 -> Mux6/1  "PhaseA"
  Demux4/2 -> IQN / IQN1/1
  Carrier1/1(Out1) -> Add18/2, Add17/2, Add16/2, Mux6/4  "PhaseN"
  Add17/1 -> Mux6/2  "PhaseB"

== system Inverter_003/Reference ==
  note: Red: Set Sample Time
  Vac Ref : Inport
  Constant10 : Constant  Value=0  OutDataTypeStr=single  SampleTime=0.1
  Constant11 : Constant  Value=0.005  OutDataTypeStr=fixdt(1,32,2^-29,0)  SampleTime=-1
  Constant13 : Constant  OutDataTypeStr=single  SampleTime=0.1
  Constant14 : Constant  Value=0  OutDataTypeStr=single  SampleTime=0.1
  Constant8 : Constant  OutDataTypeStr=fixdt(1,32,2^-29,0)  SampleTime=-1
  Constant9 : Constant  Value=0  OutDataTypeStr=fixdt(1,32,2^-29,0)  SampleTime=-1
  Float to IQN : tiiqmathlib/Float to IQN  Q_value=10
  Float to IQN1 : tiiqmathlib/Float to IQN  Q_value=10
  Float to IQN2 : tiiqmathlib/Float to IQN  Q_value=10
  Gain2 : Gain  Gain=2*pi
  Gain3 : Gain  Gain=sqrt(2)  OutDataTypeStr=Inherit: Inherit via back propagation
  IQN to Float3 : tiiqmathlib/IQN to Float
  Inverse Park Transformation : Subsystem  InitFcn=tic2000lib_licenseCheck  mask(Inverse Park Transformation){}
      mask help: This block performs vector transformation from orthogonal rotating reference frame into orthogonal stationary frame. All inputs and outputs are signed 32-bit fixed-point numbers with Q value between 1 and 29.
  Mux2 : Mux  Inputs=3
  Product5 : Product
  Ramp Generator1 : c28xdmclib/Ramp Generator  step_angle_max=1
  abc : Outport
  angle : Outport  Port=2
  dq0 : Outport  Port=3
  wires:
  Vac Ref/1 -> Gain3/1
  IQN to Float3/1 -> Gain2/1
  Constant11/1 -> Ramp Generator1/3
  Gain2/1 -> Float to IQN1/1
  Constant14/1 -> Mux2/2
  Constant9/1 -> Ramp Generator1/2
  Float to IQN2/1 -> Product5/2
  Constant10/1 -> Mux2/3
  Product5/1 -> Float to IQN/1
  Constant13/1 -> Mux2/1
  Mux2/1 -> Product5/1
  Float to IQN1/1 -> angle/1, Inverse Park Transformation/2(theta)
  Constant8/1 -> Ramp Generator1/1
  Float to IQN/1 -> dq0/1, Inverse Park Transformation/1(DQ0)
  Gain3/1 -> Float to IQN2/1
  Ramp Generator1/1 -> IQN to Float3/1
  Inverse Park Transformation/1(ABC) -> abc/1

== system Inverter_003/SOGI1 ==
  note: 1/RC
  In : Inport
  Constant : Constant  Value=2*pi*Freq
  Euler Backward : Subsystem  mask{SampleTime=SampleTime, UpperLimit=UpperLimit, LowerLimit=LowerLimit}
      mask prompts: SampleTime "Sample Time"; UpperLimit "Upper Limit"; LowerLimit "Lower Limit"
  Euler Backward1 : Subsystem  mask{SampleTime=SampleTime, UpperLimit=UpperLimit, LowerLimit=LowerLimit}
      mask prompts: SampleTime "Sample Time"; UpperLimit "Upper Limit"; LowerLimit "Lower Limit"
  Gain4 : Gain  Gain=5
  Math Function : Math  Operator=square
  Product : Product
  Sum2 : Sum  Inputs=-+|
  Sum6 : Sum  Inputs=|+-
  Unit Delay1 : UnitDelay  SampleTime=-1
  Unit Delay3 : UnitDelay  SampleTime=-1
  Out : Outport
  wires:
  Unit Delay3/1 -> Sum6/2
  Sum6/1 -> Euler Backward/1(In)
  Euler Backward1/1(Out) -> Product/1
  Constant/1 -> Math Function/1
  Euler Backward/1(Out) -> Euler Backward1/1(In), Out/1, Unit Delay1/1
  In/1 -> Sum2/2
  Product/1 -> Unit Delay3/1
  Sum2/1 -> Gain4/1
  Unit Delay1/1 -> Sum2/1
  Gain4/1 -> Sum6/1
  Math Function/1 -> Product/2
